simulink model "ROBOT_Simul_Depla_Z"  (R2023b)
settings: Solver=ode15s  StartTime=0.0  StopTime=0.2  RelTol=1e-3  EnableMultiTasking=on
undefined symbols (not defined in the file): BATI1_Défaut_sldprt, BATI2_Défaut_sldprt, BATI3_Défaut_sldprt, deg, kg, m, mm, N, rad, s, STL, X, Y, Z
libraries: sm_lib x139, fl_lib x42, nesl_utility x19, slpidlib x3
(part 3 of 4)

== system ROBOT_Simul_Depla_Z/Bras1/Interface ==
  Angular Velocity Source : fl_lib/Mechanical/Mechanical Sources/Ideal Angular Velocity Source
  Torque Sensor : fl_lib/Mechanical/Mechanical Sensors/Ideal Torque Sensor
  C : PMIOPort  Side=Left
  T : PMIOPort  Port=2  Side=Right
  w : PMIOPort  Port=3  Side=Right
  R : PMIOPort  Port=4  Side=Left
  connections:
  R/RConn1 -- Angular Velocity Source/LConn1
  Torque Sensor/LConn1 -- Angular Velocity Source/RConn2
  Torque Sensor/RConn2 -- T/RConn1
  C/RConn1 -- Torque Sensor/RConn1
  Angular Velocity Source/RConn1 -- w/RConn1

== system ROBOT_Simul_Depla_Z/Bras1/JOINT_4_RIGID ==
  ReferenceFrame : sm_lib/Frames and Transforms/Reference Frame
  Solid : sm_lib/Body Elements/File Solid  ExtGeomFileName=\STL\JOINT_Défaut_sldprt.STL  UnitType=Custom  ExtGeomFileUnits=mm  StepReaderType=HEX  ExportConvexHullGeometry=off  InertiaType=Custom  Mass=0.010425088409650831  MassUnits=kg  CenterOfMass=[-2.8413803884081348e-07 7.2198924235006832 8.2870434049836507e-08]  CenterOfMassUnits=mm  MomentsOfInertia=[0.40441054898779027 0.67355736496231777 0.88349580308055875]  MomentsOfInertiaUnits=kg*mm^2  ProductsOfInertia=[5.448486796310623e-10 1.7393207622030534e-07 1.1975376403711247e-08]  ProductsOfInertiaUnits=kg*mm^2  BasedOnType=Density  Density=1000  DensityUnits=kg/(m^3)  DoExposeReferenceFrame=on  SerializedFrames=<Frames/>  GraphicType=FromGeometry  MarkerShape=Sphere  MarkerSize=10  MarkerSizeUnits=m  GraphicVisPropType=SimpleVisualProperties  GraphicDiffuseColor=[0.792156862745098 0.81960784313725488 0.93333333333333335]  GraphicSpecularColor=[0.5 0.5 0.5 1.0]  GraphicAmbientColor=[0.15 0.15 0.15 1.0]  GraphicEmissiveColor=[0.0 0.0 0.0 1.0]  GraphicShininess=75  GraphicOpacity=1
  Transform : sm_lib/Frames and Transforms/Rigid Transform  TranslationMethod=Cartesian  TranslationStandardOffset=0  TranslationStandardOffsetUnits=mm  TranslationStandardAxis=+Z  TranslationCartesianOffset=[13.999999999999849 4.9999999999999574 4.9999999999999956]  TranslationCartesianOffsetUnits=mm  TranslationROffset=0  TranslationROffsetUnits=m  TranslationZOffset=0  TranslationZOffsetUnits=m  TranslationThetaOffset=0  TranslationThetaOffsetUnits=deg  RotationMethod=ArbitraryAxis  RotationAngleUnits=rad  RotationStandardAxis=+Z  RotationAngle=3.1415926535897931  RotationArbitraryAxis=[-1 4.2709310989463294e-33 -8.8869701386798953e-17]  FollAlignAxisA=+X  BaseAlignAxisA=+Y  FollAlignAxisB=+Y  BaseAlignAxisB=+Z  RotationSequenceAxes=FollowerAxes  RotationSequence=XYX  RotationSequenceAngles=[0 0 0]  RotationSequenceAnglesUnits=deg  RotationMatrix=[1 0 0; 0 1 0; 0 0 1]  Quaternion=[1 0 0 0]
  Transform1 : sm_lib/Frames and Transforms/Rigid Transform  TranslationMethod=Cartesian  TranslationStandardOffset=0  TranslationStandardOffsetUnits=mm  TranslationStandardAxis=+Z  TranslationCartesianOffset=[-14.000000000000142 4.9999999999998455 -4.9999999999999893]  TranslationCartesianOffsetUnits=mm  TranslationROffset=0  TranslationROffsetUnits=m  TranslationZOffset=0  TranslationZOffsetUnits=m  TranslationThetaOffset=0  TranslationThetaOffsetUnits=deg  RotationMethod=ArbitraryAxis  RotationAngleUnits=rad  RotationStandardAxis=+Z  RotationAngle=1.5700924586837749e-16  RotationArbitraryAxis=[-0.99993539825238109 0.011366587959979699 -8.9227205578830452e-19]  FollAlignAxisA=+X  BaseAlignAxisA=+Y  FollAlignAxisB=+Y  BaseAlignAxisB=+Z  RotationSequenceAxes=FollowerAxes  RotationSequence=XYX  RotationSequenceAngles=[0 0 0]  RotationSequenceAnglesUnits=deg  RotationMatrix=[1 0 0; 0 1 0; 0 0 1]  Quaternion=[1 0 0 0]
  Transform2 : sm_lib/Frames and Transforms/Rigid Transform  TranslationMethod=Cartesian  TranslationStandardOffset=0  TranslationStandardOffsetUnits=mm  TranslationStandardAxis=+Z  TranslationCartesianOffset=[-9.9999999999997335 16.250000000000529 -3.0198066269804258e-13]  TranslationCartesianOffsetUnits=mm  TranslationROffset=0  TranslationROffsetUnits=m  TranslationZOffset=0  TranslationZOffsetUnits=m  TranslationThetaOffset=0  TranslationThetaOffsetUnits=deg  RotationMethod=ArbitraryAxis  RotationAngleUnits=rad  RotationStandardAxis=+Z  RotationAngle=2.0943951023931944  RotationArbitraryAxis=[0.57735026918962729 0.57735026918962551 0.57735026918962451]  FollAlignAxisA=+X  BaseAlignAxisA=+Y  FollAlignAxisB=+Y  BaseAlignAxisB=+Z  RotationSequenceAxes=FollowerAxes  RotationSequence=XYX  RotationSequenceAngles=[0 0 0]  RotationSequenceAnglesUnits=deg  RotationMatrix=[1 0 0; 0 1 0; 0 0 1]  Quaternion=[1 0 0 0]
  F2 : PMIOPort  Side=Right
  F1 : PMIOPort  Port=2  Side=Left
  F : PMIOPort  Port=3  Side=Left
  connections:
  Solid/RConn1 -- ReferenceFrame/RConn1 -- Transform/LConn1 -- Transform1/LConn1 -- Transform2/LConn1
  Transform/RConn1 -- F/RConn1
  Transform1/RConn1 -- F1/RConn1
  Transform2/RConn1 -- F2/RConn1

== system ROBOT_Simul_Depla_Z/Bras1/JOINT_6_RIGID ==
  ReferenceFrame : sm_lib/Frames and Transforms/Reference Frame
  Solid : sm_lib/Body Elements/File Solid  ExtGeomFileName=\STL\JOINT_Défaut_sldprt.STL  UnitType=Custom  ExtGeomFileUnits=mm  StepReaderType=HEX  ExportConvexHullGeometry=off  InertiaType=Custom  Mass=0.010425088409650831  MassUnits=kg  CenterOfMass=[-2.8413803884081348e-07 7.2198924235006832 8.2870434049836507e-08]  CenterOfMassUnits=mm  MomentsOfInertia=[0.40441054898779027 0.67355736496231777 0.88349580308055875]  MomentsOfInertiaUnits=kg*mm^2  ProductsOfInertia=[5.448486796310623e-10 1.7393207622030534e-07 1.1975376403711247e-08]  ProductsOfInertiaUnits=kg*mm^2  BasedOnType=Density  Density=1000  DensityUnits=kg/(m^3)  DoExposeReferenceFrame=on  SerializedFrames=<Frames/>  GraphicType=FromGeometry  MarkerShape=Sphere  MarkerSize=10  MarkerSizeUnits=m  GraphicVisPropType=SimpleVisualProperties  GraphicDiffuseColor=[0.792156862745098 0.81960784313725488 0.93333333333333335]  GraphicSpecularColor=[0.5 0.5 0.5 1.0]  GraphicAmbientColor=[0.15 0.15 0.15 1.0]  GraphicEmissiveColor=[0.0 0.0 0.0 1.0]  GraphicShininess=75  GraphicOpacity=1
  Transform : sm_lib/Frames and Transforms/Rigid Transform  TranslationMethod=Cartesian  TranslationStandardOffset=0  TranslationStandardOffsetUnits=mm  TranslationStandardAxis=+Z  TranslationCartesianOffset=[14.000000000000327 5.0000000000000409 -4.9999999999999645]  TranslationCartesianOffsetUnits=mm  TranslationROffset=0  TranslationROffsetUnits=m  TranslationZOffset=0  TranslationZOffsetUnits=m  TranslationThetaOffset=0  TranslationThetaOffsetUnits=deg  RotationMethod=ArbitraryAxis  RotationAngleUnits=rad  RotationStandardAxis=+Z  RotationAngle=2.5476231888929306e-16  RotationArbitraryAxis=[0.25866689172319263 0.96596658282068038 3.1827911693718406e-17]  FollAlignAxisA=+X  BaseAlignAxisA=+Y  FollAlignAxisB=+Y  BaseAlignAxisB=+Z  RotationSequenceAxes=FollowerAxes  RotationSequence=XYX  RotationSequenceAngles=[0 0 0]  RotationSequenceAnglesUnits=deg  RotationMatrix=[1 0 0; 0 1 0; 0 0 1]  Quaternion=[1 0 0 0]
  Transform1 : sm_lib/Frames and Transforms/Rigid Transform  TranslationMethod=Cartesian  TranslationStandardOffset=0  TranslationStandardOffsetUnits=mm  TranslationStandardAxis=+Z  TranslationCartesianOffset=[-13.999999999999677 5.0000000000000444 4.9999999999999964]  TranslationCartesianOffsetUnits=mm  TranslationROffset=0  TranslationROffsetUnits=m  TranslationZOffset=0  TranslationZOffsetUnits=m  TranslationThetaOffset=0  TranslationThetaOffsetUnits=deg  RotationMethod=ArbitraryAxis  RotationAngleUnits=rad  RotationStandardAxis=+Z  RotationAngle=3.1415926535897931  RotationArbitraryAxis=[1 -6.1548272841853811e-33 -8.2569214265266672e-17]  FollAlignAxisA=+X  BaseAlignAxisA=+Y  FollAlignAxisB=+Y  BaseAlignAxisB=+Z  RotationSequenceAxes=FollowerAxes  RotationSequence=XYX  RotationSequenceAngles=[0 0 0]  RotationSequenceAnglesUnits=deg  RotationMatrix=[1 0 0; 0 1 0; 0 0 1]  Quaternion=[1 0 0 0]
  Transform2 : sm_lib/Frames and Transforms/Rigid Transform  TranslationMethod=Cartesian  TranslationStandardOffset=0  TranslationStandardOffsetUnits=mm  TranslationStandardAxis=+Z  TranslationCartesianOffset=[10.000000000006413 16.249999999997939 -2.3288038164537284e-12]  TranslationCartesianOffsetUnits=mm  TranslationROffset=0  TranslationROffsetUnits=m  TranslationZOffset=0  TranslationZOffsetUnits=m  TranslationThetaOffset=0  TranslationThetaOffsetUnits=deg  RotationMethod=ArbitraryAxis  RotationAngleUnits=rad  RotationStandardAxis=+Z  RotationAngle=2.0943951023931966  RotationArbitraryAxis=[-0.5773502691896264 -0.57735026918962618 0.57735026918962484]  FollAlignAxisA=+X  BaseAlignAxisA=+Y  FollAlignAxisB=+Y  BaseAlignAxisB=+Z  RotationSequenceAxes=FollowerAxes  RotationSequence=XYX  RotationSequenceAngles=[0 0 0]  RotationSequenceAnglesUnits=deg  RotationMatrix=[1 0 0; 0 1 0; 0 0 1]  Quaternion=[1 0 0 0]
  F2 : PMIOPort  Side=Left
  F1 : PMIOPort  Port=2  Side=Right
  F : PMIOPort  Port=3  Side=Right
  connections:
  Solid/RConn1 -- ReferenceFrame/RConn1 -- Transform/LConn1 -- Transform1/LConn1 -- Transform2/LConn1
  Transform/RConn1 -- F/RConn1
  Transform1/RConn1 -- F1/RConn1
  Transform2/RConn1 -- F2/RConn1

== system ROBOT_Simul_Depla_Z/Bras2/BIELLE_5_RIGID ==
  ReferenceFrame : sm_lib/Frames and Transforms/Reference Frame
  Solid : sm_lib/Body Elements/File Solid  ExtGeomFileName=\STL\BIELLE_Défaut_sldprt.STL  UnitType=Custom  ExtGeomFileUnits=mm  StepReaderType=HEX  ExportConvexHullGeometry=off  InertiaType=Custom  Mass=0.008350539405564527  MassUnits=kg  CenterOfMass=[0 1.3968069938607398e-07 -5.4963035279888423e-06]  CenterOfMassUnits=mm  MomentsOfInertia=[9.7237898508136684 9.7147278737202658 0.035523108889582884]  MomentsOfInertiaUnits=kg*mm^2  ProductsOfInertia=[0 -4.4011490170351759e-08 -8.1673382975267321e-07]  ProductsOfInertiaUnits=kg*mm^2  BasedOnType=Density  Density=1000  DensityUnits=kg/(m^3)  DoExposeReferenceFrame=on  SerializedFrames=<Frames/>  GraphicType=FromGeometry  MarkerShape=Sphere  MarkerSize=10  MarkerSizeUnits=m  GraphicVisPropType=SimpleVisualProperties  GraphicDiffuseColor=[0.69803921568627447 0.69803921568627447 0.69803921568627447]  GraphicSpecularColor=[0.5 0.5 0.5 1.0]  GraphicAmbientColor=[0.15 0.15 0.15 1.0]  GraphicEmissiveColor=[0.0 0.0 0.0 1.0]  GraphicShininess=75  GraphicOpacity=1
  Transform : sm_lib/Frames and Transforms/Rigid Transform  TranslationMethod=Cartesian  TranslationStandardOffset=0  TranslationStandardOffsetUnits=mm  TranslationStandardAxis=+Z  TranslationCartesianOffset=[0 4.9999999999999973 -51.250000000000007]  TranslationCartesianOffsetUnits=mm  TranslationROffset=0  TranslationROffsetUnits=m  TranslationZOffset=0  TranslationZOffsetUnits=m  TranslationThetaOffset=0  TranslationThetaOffsetUnits=deg  RotationMethod=ArbitraryAxis  RotationAngleUnits=rad  RotationStandardAxis=+Z  RotationAngle=2.0943951023931953  RotationArbitraryAxis=[0.57735026918962584 -0.57735026918962584 0.57735026918962584]  FollAlignAxisA=+X  BaseAlignAxisA=+Y  FollAlignAxisB=+Y  BaseAlignAxisB=+Z  RotationSequenceAxes=FollowerAxes  RotationSequence=XYX  RotationSequenceAngles=[0 0 0]  RotationSequenceAnglesUnits=deg  RotationMatrix=[1 0 0; 0 1 0; 0 0 1]  Quaternion=[1 0 0 0]
  Transform1 : sm_lib/Frames and Transforms/Rigid Transform  TranslationMethod=Cartesian  TranslationStandardOffset=0  TranslationStandardOffsetUnits=mm  TranslationStandardAxis=+Z  TranslationCartesianOffset=[0 5.0000000000000044 51.249999999999993]  TranslationCartesianOffsetUnits=mm  TranslationROffset=0  TranslationROffsetUnits=m  TranslationZOffset=0  TranslationZOffsetUnits=m  TranslationThetaOffset=0  TranslationThetaOffsetUnits=deg  RotationMethod=ArbitraryAxis  RotationAngleUnits=rad  RotationStandardAxis=+Z  RotationAngle=2.0943951023931953  RotationArbitraryAxis=[0.57735026918962584 -0.57735026918962584 0.57735026918962584]  FollAlignAxisA=+X  BaseAlignAxisA=+Y  FollAlignAxisB=+Y  BaseAlignAxisB=+Z  RotationSequenceAxes=FollowerAxes  RotationSequence=XYX  RotationSequenceAngles=[0 0 0]  RotationSequenceAnglesUnits=deg  RotationMatrix=[1 0 0; 0 1 0; 0 0 1]  Quaternion=[1 0 0 0]
  F : PMIOPort  Side=Left
  F1 : PMIOPort  Port=2  Side=Right
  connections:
  Solid/RConn1 -- ReferenceFrame/RConn1 -- Transform/LConn1 -- Transform1/LConn1
  Transform/RConn1 -- F/RConn1
  Transform1/RConn1 -- F1/RConn1

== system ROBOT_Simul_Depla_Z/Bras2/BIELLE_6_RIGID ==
  ReferenceFrame : sm_lib/Frames and Transforms/Reference Frame
  Solid : sm_lib/Body Elements/File Solid  ExtGeomFileName=\STL\BIELLE_Défaut_sldprt.STL  UnitType=Custom  ExtGeomFileUnits=mm  StepReaderType=HEX  ExportConvexHullGeometry=off  InertiaType=Custom  Mass=0.008350539405564527  MassUnits=kg  CenterOfMass=[0 1.3968069938607398e-07 -5.4963035279888423e-06]  CenterOfMassUnits=mm  MomentsOfInertia=[9.7237898508136684 9.7147278737202658 0.035523108889582884]  MomentsOfInertiaUnits=kg*mm^2  ProductsOfInertia=[0 -4.4011490170351759e-08 -8.1673382975267321e-07]  ProductsOfInertiaUnits=kg*mm^2  BasedOnType=Density  Density=1000  DensityUnits=kg/(m^3)  DoExposeReferenceFrame=on  SerializedFrames=<Frames/>  GraphicType=FromGeometry  MarkerShape=Sphere  MarkerSize=10  MarkerSizeUnits=m  GraphicVisPropType=SimpleVisualProperties  GraphicDiffuseColor=[0.69803921568627447 0.69803921568627447 0.69803921568627447]  GraphicSpecularColor=[0.5 0.5 0.5 1.0]  GraphicAmbientColor=[0.15 0.15 0.15 1.0]  GraphicEmissiveColor=[0.0 0.0 0.0 1.0]  GraphicShininess=75  GraphicOpacity=1
  Transform : sm_lib/Frames and Transforms/Rigid Transform  TranslationMethod=Cartesian  TranslationStandardOffset=0  TranslationStandardOffsetUnits=mm  TranslationStandardAxis=+Z  TranslationCartesianOffset=[0 4.9999999999999902 -51.249999999999993]  TranslationCartesianOffsetUnits=mm  TranslationROffset=0  TranslationROffsetUnits=m  TranslationZOffset=0  TranslationZOffsetUnits=m  TranslationThetaOffset=0  TranslationThetaOffsetUnits=deg  RotationMethod=ArbitraryAxis  RotationAngleUnits=rad  RotationStandardAxis=+Z  RotationAngle=2.0943951023931953  RotationArbitraryAxis=[0.57735026918962584 -0.57735026918962584 0.57735026918962584]  FollAlignAxisA=+X  BaseAlignAxisA=+Y  FollAlignAxisB=+Y  BaseAlignAxisB=+Z  RotationSequenceAxes=FollowerAxes  RotationSequence=XYX  RotationSequenceAngles=[0 0 0]  RotationSequenceAnglesUnits=deg  RotationMatrix=[1 0 0; 0 1 0; 0 0 1]  Quaternion=[1 0 0 0]
  Transform1 : sm_lib/Frames and Transforms/Rigid Transform  TranslationMethod=Cartesian  TranslationStandardOffset=0  TranslationStandardOffsetUnits=mm  TranslationStandardAxis=+Z  TranslationCartesianOffset=[0 4.9999999999999902 51.25]  TranslationCartesianOffsetUnits=mm  TranslationROffset=0  TranslationROffsetUnits=m  TranslationZOffset=0  TranslationZOffsetUnits=m  TranslationThetaOffset=0  TranslationThetaOffsetUnits=deg  RotationMethod=ArbitraryAxis  RotationAngleUnits=rad  RotationStandardAxis=+Z  RotationAngle=2.0943951023931953  RotationArbitraryAxis=[0.57735026918962584 -0.57735026918962584 0.57735026918962584]  FollAlignAxisA=+X  BaseAlignAxisA=+Y  FollAlignAxisB=+Y  BaseAlignAxisB=+Z  RotationSequenceAxes=FollowerAxes  RotationSequence=XYX  RotationSequenceAngles=[0 0 0]  RotationSequenceAnglesUnits=deg  RotationMatrix=[1 0 0; 0 1 0; 0 0 1]  Quaternion=[1 0 0 0]
  F : PMIOPort  Side=Left
  F1 : PMIOPort  Port=2  Side=Right
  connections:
  Solid/RConn1 -- ReferenceFrame/RConn1 -- Transform/LConn1 -- Transform1/LConn1
  Transform/RConn1 -- F/RConn1
  Transform1/RConn1 -- F1/RConn1

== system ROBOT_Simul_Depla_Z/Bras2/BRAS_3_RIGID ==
  BRAS_1_RIGID : Subsystem
  BRAS_3_RIGID : Subsystem
  ReferenceFrame : sm_lib/Frames and Transforms/Reference Frame
  Transform : sm_lib/Frames and Transforms/Rigid Transform  TranslationMethod=Cartesian  TranslationStandardOffset=0  TranslationStandardOffsetUnits=mm  TranslationStandardAxis=+Z  TranslationCartesianOffset=[-7.3896444519050419e-13 -16.842456388464797 5.0000000000063061]  TranslationCartesianOffsetUnits=mm  TranslationROffset=0  TranslationROffsetUnits=m  TranslationZOffset=0  TranslationZOffsetUnits=m  TranslationThetaOffset=0  TranslationThetaOffsetUnits=deg  RotationMethod=ArbitraryAxis  RotationAngleUnits=rad  RotationStandardAxis=+Z  RotationAngle=3.1415926535897922  RotationArbitraryAxis=[1 -3.4968219954323673e-31 -7.4654377952851924e-16]  FollAlignAxisA=+X  BaseAlignAxisA=+Y  FollAlignAxisB=+Y  BaseAlignAxisB=+Z  RotationSequenceAxes=FollowerAxes  RotationSequence=XYX  RotationSequenceAngles=[0 0 0]  RotationSequenceAnglesUnits=deg  RotationMatrix=[1 0 0; 0 1 0; 0 0 1]  Quaternion=[1 0 0 0]
  Transform1 : sm_lib/Frames and Transforms/Rigid Transform  TranslationMethod=Cartesian  TranslationStandardOffset=0  TranslationStandardOffsetUnits=mm  TranslationStandardAxis=+Z  TranslationCartesianOffset=[0 43.157543611535338 10.000000000006285]  TranslationCartesianOffsetUnits=mm  TranslationROffset=0  TranslationROffsetUnits=m  TranslationZOffset=0  TranslationZOffsetUnits=m  TranslationThetaOffset=0  TranslationThetaOffsetUnits=deg  RotationMethod=ArbitraryAxis  RotationAngleUnits=rad  RotationStandardAxis=+Z  RotationAngle=3.1415926535897931  RotationArbitraryAxis=[1 0 0]  FollAlignAxisA=+X  BaseAlignAxisA=+Y  FollAlignAxisB=+Y  BaseAlignAxisB=+Z  RotationSequenceAxes=FollowerAxes  RotationSequence=XYX  RotationSequenceAngles=[0 0 0]  RotationSequenceAnglesUnits=deg  RotationMatrix=[1 0 0; 0 1 0; 0 0 1]  Quaternion=[1 0 0 0]
  Transform2 : sm_lib/Frames and Transforms/Rigid Transform  TranslationMethod=Cartesian  TranslationStandardOffset=0  TranslationStandardOffsetUnits=mm  TranslationStandardAxis=+Z  TranslationCartesianOffset=[0 -16.842456388464662 6.2762295360840881e-12]  TranslationCartesianOffsetUnits=mm  TranslationROffset=0  TranslationROffsetUnits=m  TranslationZOffset=0  TranslationZOffsetUnits=m  TranslationThetaOffset=0  TranslationThetaOffsetUnits=deg  RotationMethod=None  RotationAngleUnits=deg  RotationStandardAxis=+Z  RotationAngle=0  RotationArbitraryAxis=[0 0 1]  FollAlignAxisA=+X  BaseAlignAxisA=+Y  FollAlignAxisB=+Y  BaseAlignAxisB=+Z  RotationSequenceAxes=FollowerAxes  RotationSequence=XYX  RotationSequenceAngles=[0 0 0]  RotationSequenceAnglesUnits=deg  RotationMatrix=[1 0 0; 0 1 0; 0 0 1]  Quaternion=[1 0 0 0]
  Transform3 : sm_lib/Frames and Transforms/Rigid Transform  TranslationMethod=Cartesian  TranslationStandardOffset=0  TranslationStandardOffsetUnits=mm  TranslationStandardAxis=+Z  TranslationCartesianOffset=[0 43.157543611535338 6.2692906421801808e-12]  TranslationCartesianOffsetUnits=mm  TranslationROffset=0  TranslationROffsetUnits=m  TranslationZOffset=0  TranslationZOffsetUnits=m  TranslationThetaOffset=0  TranslationThetaOffsetUnits=deg  RotationMethod=ArbitraryAxis  RotationAngleUnits=rad  RotationStandardAxis=+Z  RotationAngle=3.1415926535897931  RotationArbitraryAxis=[0 0 1]  FollAlignAxisA=+X  BaseAlignAxisA=+Y  FollAlignAxisB=+Y  BaseAlignAxisB=+Z  RotationSequenceAxes=FollowerAxes  RotationSequence=XYX  RotationSequenceAngles=[0 0 0]  RotationSequenceAnglesUnits=deg  RotationMatrix=[1 0 0; 0 1 0; 0 0 1]  Quaternion=[1 0 0 0]
  F : PMIOPort  Side=Left
  F1 : PMIOPort  Port=2  Side=Right
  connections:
  Transform/LConn1 -- ReferenceFrame/RConn1 -- Transform1/LConn1 -- Transform2/LConn1 -- Transform3/LConn1
  Transform/RConn1 -- F/RConn1
  Transform1/RConn1 -- F1/RConn1
  BRAS_1_RIGID/LConn1 -- Transform2/RConn1
  BRAS_3_RIGID/LConn1 -- Transform3/RConn1

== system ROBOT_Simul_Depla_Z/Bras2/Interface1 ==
  Angular Velocity Source : fl_lib/Mechanical/Mechanical Sources/Ideal Angular Velocity Source
  Torque Sensor : fl_lib/Mechanical/Mechanical Sensors/Ideal Torque Sensor
  C : PMIOPort  Side=Left
  T : PMIOPort  Port=2  Side=Right
  w : PMIOPort  Port=3  Side=Right
  R : PMIOPort  Port=4  Side=Left
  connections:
  Angular Velocity Source/RConn1 -- w/RConn1
  C/RConn1 -- Torque Sensor/RConn1
  Torque Sensor/RConn2 -- T/RConn1
  Torque Sensor/LConn1 -- Angular Velocity Source/RConn2
  R/RConn1 -- Angular Velocity Source/LConn1

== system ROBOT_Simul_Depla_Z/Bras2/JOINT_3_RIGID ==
  ReferenceFrame : sm_lib/Frames and Transforms/Reference Frame
  Solid : sm_lib/Body Elements/File Solid  ExtGeomFileName=\STL\JOINT_Défaut_sldprt.STL  UnitType=Custom  ExtGeomFileUnits=mm  StepReaderType=HEX  ExportConvexHullGeometry=off  InertiaType=Custom  Mass=0.010425088409650831  MassUnits=kg  CenterOfMass=[-2.8413803884081348e-07 7.2198924235006832 8.2870434049836507e-08]  CenterOfMassUnits=mm  MomentsOfInertia=[0.40441054898779027 0.67355736496231777 0.88349580308055875]  MomentsOfInertiaUnits=kg*mm^2  ProductsOfInertia=[5.448486796310623e-10 1.7393207622030534e-07 1.1975376403711247e-08]  ProductsOfInertiaUnits=kg*mm^2  BasedOnType=Density  Density=1000  DensityUnits=kg/(m^3)  DoExposeReferenceFrame=on  SerializedFrames=<Frames/>  GraphicType=FromGeometry  MarkerShape=Sphere  MarkerSize=10  MarkerSizeUnits=m  GraphicVisPropType=SimpleVisualProperties  GraphicDiffuseColor=[0.792156862745098 0.81960784313725488 0.93333333333333335]  GraphicSpecularColor=[0.5 0.5 0.5 1.0]  GraphicAmbientColor=[0.15 0.15 0.15 1.0]  GraphicEmissiveColor=[0.0 0.0 0.0 1.0]  GraphicShininess=75  GraphicOpacity=1
  Transform : sm_lib/Frames and Transforms/Rigid Transform  TranslationMethod=Cartesian  TranslationStandardOffset=0  TranslationStandardOffsetUnits=mm  TranslationStandardAxis=+Z  TranslationCartesianOffset=[14.000000000000393 5.0000000000002949 4.9999999999999307]  TranslationCartesianOffsetUnits=mm  TranslationROffset=0  TranslationROffsetUnits=m  TranslationZOffset=0  TranslationZOffsetUnits=m  TranslationThetaOffset=0  TranslationThetaOffsetUnits=deg  RotationMethod=ArbitraryAxis  RotationAngleUnits=rad  RotationStandardAxis=+Z  RotationAngle=3.1415926535897927  RotationArbitraryAxis=[1 2.4716035461156956e-31 6.8614764825058098e-16]  FollAlignAxisA=+X  BaseAlignAxisA=+Y  FollAlignAxisB=+Y  BaseAlignAxisB=+Z  RotationSequenceAxes=FollowerAxes  RotationSequence=XYX  RotationSequenceAngles=[0 0 0]  RotationSequenceAnglesUnits=deg  RotationMatrix=[1 0 0; 0 1 0; 0 0 1]  Quaternion=[1 0 0 0]
  Transform1 : sm_lib/Frames and Transforms/Rigid Transform  TranslationMethod=Cartesian  TranslationStandardOffset=0  TranslationStandardOffsetUnits=mm  TranslationStandardAxis=+Z  TranslationCartesianOffset=[-13.999999999999581 5.0000000000001972 4.9999999999999769]  TranslationCartesianOffsetUnits=mm  TranslationROffset=0  TranslationROffsetUnits=m  TranslationZOffset=0  TranslationZOffsetUnits=m  TranslationThetaOffset=0  TranslationThetaOffsetUnits=deg  RotationMethod=ArbitraryAxis  RotationAngleUnits=rad  RotationStandardAxis=+Z  RotationAngle=3.1415926535897931  RotationArbitraryAxis=[1 6.1605098685514057e-33 4.1234572726680469e-16]  FollAlignAxisA=+X  BaseAlignAxisA=+Y  FollAlignAxisB=+Y  BaseAlignAxisB=+Z  RotationSequenceAxes=FollowerAxes  RotationSequence=XYX  RotationSequenceAngles=[0 0 0]  RotationSequenceAnglesUnits=deg  RotationMatrix=[1 0 0; 0 1 0; 0 0 1]  Quaternion=[1 0 0 0]
  Transform2 : sm_lib/Frames and Transforms/Rigid Transform  TranslationMethod=Cartesian  TranslationStandardOffset=0  TranslationStandardOffsetUnits=mm  TranslationStandardAxis=+Z  TranslationCartesianOffset=[-10.000000000000021 16.250000000001698 1.8616219676914625e-12]  TranslationCartesianOffsetUnits=mm  TranslationROffset=0  TranslationROffsetUnits=m  TranslationZOffset=0  TranslationZOffsetUnits=m  TranslationThetaOffset=0  TranslationThetaOffsetUnits=deg  RotationMethod=ArbitraryAxis  RotationAngleUnits=rad  RotationStandardAxis=+Z  RotationAngle=2.0943951023931962  RotationArbitraryAxis=[0.57735026918962506 0.57735026918962606 0.57735026918962606]  FollAlignAxisA=+X  BaseAlignAxisA=+Y  FollAlignAxisB=+Y  BaseAlignAxisB=+Z  RotationSequenceAxes=FollowerAxes  RotationSequence=XYX  RotationSequenceAngles=[0 0 0]  RotationSequenceAnglesUnits=deg  RotationMatrix=[1 0 0; 0 1 0; 0 0 1]  Quaternion=[1 0 0 0]
  F2 : PMIOPort  Side=Left
  F1 : PMIOPort  Port=2  Side=Right
  F : PMIOPort  Port=3  Side=Right
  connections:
  Solid/RConn1 -- ReferenceFrame/RConn1 -- Transform/LConn1 -- Transform1/LConn1 -- Transform2/LConn1
  Transform/RConn1 -- F/RConn1
  Transform1/RConn1 -- F1/RConn1
  Transform2/RConn1 -- F2/RConn1

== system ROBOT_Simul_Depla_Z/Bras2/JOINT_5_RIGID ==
  ReferenceFrame : sm_lib/Frames and Transforms/Reference Frame
  Solid : sm_lib/Body Elements/File Solid  ExtGeomFileName=\STL\JOINT_Défaut_sldprt.STL  UnitType=Custom  ExtGeomFileUnits=mm  StepReaderType=HEX  ExportConvexHullGeometry=off  InertiaType=Custom  Mass=0.010425088409650831  MassUnits=kg  CenterOfMass=[-2.8413803884081348e-07 7.2198924235006832 8.2870434049836507e-08]  CenterOfMassUnits=mm  MomentsOfInertia=[0.40441054898779027 0.67355736496231777 0.88349580308055875]  MomentsOfInertiaUnits=kg*mm^2  ProductsOfInertia=[5.448486796310623e-10 1.7393207622030534e-07 1.1975376403711247e-08]  ProductsOfInertiaUnits=kg*mm^2  BasedOnType=Density  Density=1000  DensityUnits=kg/(m^3)  DoExposeReferenceFrame=on  SerializedFrames=<Frames/>  GraphicType=FromGeometry  MarkerShape=Sphere  MarkerSize=10  MarkerSizeUnits=m  GraphicVisPropType=SimpleVisualProperties  GraphicDiffuseColor=[0.792156862745098 0.81960784313725488 0.93333333333333335]  GraphicSpecularColor=[0.5 0.5 0.5 1.0]  GraphicAmbientColor=[0.15 0.15 0.15 1.0]  GraphicEmissiveColor=[0.0 0.0 0.0 1.0]  GraphicShininess=75  GraphicOpacity=1
  Transform : sm_lib/Frames and Transforms/Rigid Transform  TranslationMethod=Cartesian  TranslationStandardOffset=0  TranslationStandardOffsetUnits=mm  TranslationStandardAxis=+Z  TranslationCartesianOffset=[-13.99999999999973 4.9999999999999307 4.9999999999999662]  TranslationCartesianOffsetUnits=mm  TranslationROffset=0  TranslationROffsetUnits=m  TranslationZOffset=0  TranslationZOffsetUnits=m  TranslationThetaOffset=0  TranslationThetaOffsetUnits=deg  RotationMethod=ArbitraryAxis  RotationAngleUnits=rad  RotationStandardAxis=+Z  RotationAngle=3.1415926535897931  RotationArbitraryAxis=[-1 -6.4240613722994368e-33 4.1034435102868363e-17]  FollAlignAxisA=+X  BaseAlignAxisA=+Y  FollAlignAxisB=+Y  BaseAlignAxisB=+Z  RotationSequenceAxes=FollowerAxes  RotationSequence=XYX  RotationSequenceAngles=[0 0 0]  RotationSequenceAnglesUnits=deg  RotationMatrix=[1 0 0; 0 1 0; 0 0 1]  Quaternion=[1 0 0 0]
  Transform1 : sm_lib/Frames and Transforms/Rigid Transform  TranslationMethod=Cartesian  TranslationStandardOffset=0  TranslationStandardOffsetUnits=mm  TranslationStandardAxis=+Z  TranslationCartesianOffset=[14.000000000000249 4.9999999999997691 4.9999999999999734]  TranslationCartesianOffsetUnits=mm  TranslationROffset=0  TranslationROffsetUnits=m  TranslationZOffset=0  TranslationZOffsetUnits=m  TranslationThetaOffset=0  TranslationThetaOffsetUnits=deg  RotationMethod=ArbitraryAxis  RotationAngleUnits=rad  RotationStandardAxis=+Z  RotationAngle=3.1415926535897927  RotationArbitraryAxis=[1 5.1356244409297584e-32 2.9638105957297091e-16]  FollAlignAxisA=+X  BaseAlignAxisA=+Y  FollAlignAxisB=+Y  BaseAlignAxisB=+Z  RotationSequenceAxes=FollowerAxes  RotationSequence=XYX  RotationSequenceAngles=[0 0 0]  RotationSequenceAnglesUnits=deg  RotationMatrix=[1 0 0; 0 1 0; 0 0 1]  Quaternion=[1 0 0 0]
  Transform2 : sm_lib/Frames and Transforms/Rigid Transform  TranslationMethod=Cartesian  TranslationStandardOffset=0  TranslationStandardOffsetUnits=mm  TranslationStandardAxis=+Z  TranslationCartesianOffset=[10.000000000000179 16.249999999999421 -3.836930773104541e-13]  TranslationCartesianOffsetUnits=mm  TranslationROffset=0  TranslationROffsetUnits=m  TranslationZOffset=0  TranslationZOffsetUnits=m  TranslationThetaOffset=0  TranslationThetaOffsetUnits=deg  RotationMethod=ArbitraryAxis  RotationAngleUnits=rad  RotationStandardAxis=+Z  RotationAngle=2.0943951023931962  RotationArbitraryAxis=[-0.57735026918962651 -0.57735026918962606 0.57735026918962473]  FollAlignAxisA=+X  BaseAlignAxisA=+Y  FollAlignAxisB=+Y  BaseAlignAxisB=+Z  RotationSequenceAxes=FollowerAxes  RotationSequence=XYX  RotationSequenceAngles=[0 0 0]  RotationSequenceAnglesUnits=deg  RotationMatrix=[1 0 0; 0 1 0; 0 0 1]  Quaternion=[1 0 0 0]
  F1 : PMIOPort  Side=Left
  F : PMIOPort  Port=2  Side=Left
  F2 : PMIOPort  Port=3  Side=Right
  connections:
  Solid/RConn1 -- ReferenceFrame/RConn1 -- Transform/LConn1 -- Transform1/LConn1 -- Transform2/LConn1
  Transform/RConn1 -- F/RConn1
  Transform1/RConn1 -- F1/RConn1
  Transform2/RConn1 -- F2/RConn1

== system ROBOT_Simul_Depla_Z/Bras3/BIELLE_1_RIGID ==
  ReferenceFrame : sm_lib/Frames and Transforms/Reference Frame
  Solid : sm_lib/Body Elements/File Solid  ExtGeomFileName=\STL\BIELLE_Défaut_sldprt.STL  UnitType=Custom  ExtGeomFileUnits=mm  StepReaderType=HEX  ExportConvexHullGeometry=off  InertiaType=Custom  Mass=0.008350539405564527  MassUnits=kg  CenterOfMass=[0 1.3968069938607398e-07 -5.4963035279888423e-06]  CenterOfMassUnits=mm  MomentsOfInertia=[9.7237898508136684 9.7147278737202658 0.035523108889582884]  MomentsOfInertiaUnits=kg*mm^2  ProductsOfInertia=[0 -4.4011490170351759e-08 -8.1673382975267321e-07]  ProductsOfInertiaUnits=kg*mm^2  BasedOnType=Density  Density=1000  DensityUnits=kg/(m^3)  DoExposeReferenceFrame=on  SerializedFrames=<Frames/>  GraphicType=FromGeometry  MarkerShape=Sphere  MarkerSize=10  MarkerSizeUnits=m  GraphicVisPropType=SimpleVisualProperties  GraphicDiffuseColor=[0.69803921568627447 0.69803921568627447 0.69803921568627447]  GraphicSpecularColor=[0.5 0.5 0.5 1.0]  GraphicAmbientColor=[0.15 0.15 0.15 1.0]  GraphicEmissiveColor=[0.0 0.0 0.0 1.0]  GraphicShininess=75  GraphicOpacity=1
  Transform : sm_lib/Frames and Transforms/Rigid Transform  TranslationMethod=Cartesian  TranslationStandardOffset=0  TranslationStandardOffsetUnits=mm  TranslationStandardAxis=+Z  TranslationCartesianOffset=[6.4659388954169117e-13 -4.9999999999998401 -51.250000000000263]  TranslationCartesianOffsetUnits=mm  TranslationROffset=0  TranslationROffsetUnits=m  TranslationZOffset=0  TranslationZOffsetUnits=m  TranslationThetaOffset=0  TranslationThetaOffsetUnits=deg  RotationMethod=ArbitraryAxis  RotationAngleUnits=rad  RotationStandardAxis=+Z  RotationAngle=2.0943951023931953  RotationArbitraryAxis=[-0.57735026918962584 -0.57735026918962584 -0.57735026918962584]  FollAlignAxisA=+X  BaseAlignAxisA=+Y  FollAlignAxisB=+Y  BaseAlignAxisB=+Z  RotationSequenceAxes=FollowerAxes  RotationSequence=XYX  RotationSequenceAngles=[0 0 0]  RotationSequenceAnglesUnits=deg  RotationMatrix=[1 0 0; 0 1 0; 0 0 1]  Quaternion=[1 0 0 0]
  Transform1 : sm_lib/Frames and Transforms/Rigid Transform  TranslationMethod=Cartesian  TranslationStandardOffset=0  TranslationStandardOffsetUnits=mm  TranslationStandardAxis=+Z  TranslationCartesianOffset=[0 4.9999999999999973 51.249999999999986]  TranslationCartesianOffsetUnits=mm  TranslationROffset=0  TranslationROffsetUnits=m  TranslationZOffset=0  TranslationZOffsetUnits=m  TranslationThetaOffset=0  TranslationThetaOffsetUnits=deg  RotationMethod=ArbitraryAxis  RotationAngleUnits=rad  RotationStandardAxis=+Z  RotationAngle=2.0943951023931953  RotationArbitraryAxis=[0.57735026918962584 -0.57735026918962584 0.57735026918962584]  FollAlignAxisA=+X  BaseAlignAxisA=+Y  FollAlignAxisB=+Y  BaseAlignAxisB=+Z  RotationSequenceAxes=FollowerAxes  RotationSequence=XYX  RotationSequenceAngles=[0 0 0]  RotationSequenceAnglesUnits=deg  RotationMatrix=[1 0 0; 0 1 0; 0 0 1]  Quaternion=[1 0 0 0]
  F : PMIOPort  Side=Left
  F1 : PMIOPort  Port=2  Side=Right
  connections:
  Solid/RConn1 -- ReferenceFrame/RConn1 -- Transform/LConn1 -- Transform1/LConn1
  Transform/RConn1 -- F/RConn1
  Transform1/RConn1 -- F1/RConn1

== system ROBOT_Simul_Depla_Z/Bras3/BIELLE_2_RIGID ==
  ReferenceFrame : sm_lib/Frames and Transforms/Reference Frame
  Solid : sm_lib/Body Elements/File Solid  ExtGeomFileName=\STL\BIELLE_Défaut_sldprt.STL  UnitType=Custom  ExtGeomFileUnits=mm  StepReaderType=HEX  ExportConvexHullGeometry=off  InertiaType=Custom  Mass=0.008350539405564527  MassUnits=kg  CenterOfMass=[0 1.3968069938607398e-07 -5.4963035279888423e-06]  CenterOfMassUnits=mm  MomentsOfInertia=[9.7237898508136684 9.7147278737202658 0.035523108889582884]  MomentsOfInertiaUnits=kg*mm^2  ProductsOfInertia=[0 -4.4011490170351759e-08 -8.1673382975267321e-07]  ProductsOfInertiaUnits=kg*mm^2  BasedOnType=Density  Density=1000  DensityUnits=kg/(m^3)  DoExposeReferenceFrame=on  SerializedFrames=<Frames/>  GraphicType=FromGeometry  MarkerShape=Sphere  MarkerSize=10  MarkerSizeUnits=m  GraphicVisPropType=SimpleVisualProperties  GraphicDiffuseColor=[0.69803921568627447 0.69803921568627447 0.69803921568627447]  GraphicSpecularColor=[0.5 0.5 0.5 1.0]  GraphicAmbientColor=[0.15 0.15 0.15 1.0]  GraphicEmissiveColor=[0.0 0.0 0.0 1.0]  GraphicShininess=75  GraphicOpacity=1
  Transform : sm_lib/Frames and Transforms/Rigid Transform  TranslationMethod=Cartesian  TranslationStandardOffset=0  TranslationStandardOffsetUnits=mm  TranslationStandardAxis=+Z  TranslationCartesianOffset=[-6.5369931689929217e-13 -5.0000000000000746 51.250000000000604]  TranslationCartesianOffsetUnits=mm  TranslationROffset=0  TranslationROffsetUnits=m  TranslationZOffset=0  TranslationZOffsetUnits=m  TranslationThetaOffset=0  TranslationThetaOffsetUnits=deg  RotationMethod=ArbitraryAxis  RotationAngleUnits=rad  RotationStandardAxis=+Z  RotationAngle=2.0943951023931944  RotationArbitraryAxis=[-0.5773502691896254 -0.57735026918962551 -0.5773502691896264]  FollAlignAxisA=+X  BaseAlignAxisA=+Y  FollAlignAxisB=+Y  BaseAlignAxisB=+Z  RotationSequenceAxes=FollowerAxes  RotationSequence=XYX  RotationSequenceAngles=[0 0 0]  RotationSequenceAnglesUnits=deg  RotationMatrix=[1 0 0; 0 1 0; 0 0 1]  Quaternion=[1 0 0 0]
  Transform1 : sm_lib/Frames and Transforms/Rigid Transform  TranslationMethod=Cartesian  TranslationStandardOffset=0  TranslationStandardOffsetUnits=mm  TranslationStandardAxis=+Z  TranslationCartesianOffset=[0 4.9999999999999902 -51.250000000000007]  TranslationCartesianOffsetUnits=mm  TranslationROffset=0  TranslationROffsetUnits=m  TranslationZOffset=0  TranslationZOffsetUnits=m  TranslationThetaOffset=0  TranslationThetaOffsetUnits=deg  RotationMethod=ArbitraryAxis  RotationAngleUnits=rad  RotationStandardAxis=+Z  RotationAngle=2.0943951023931953  RotationArbitraryAxis=[0.57735026918962584 -0.57735026918962584 0.57735026918962584]  FollAlignAxisA=+X  BaseAlignAxisA=+Y  FollAlignAxisB=+Y  BaseAlignAxisB=+Z  RotationSequenceAxes=FollowerAxes  RotationSequence=XYX  RotationSequenceAngles=[0 0 0]  RotationSequenceAnglesUnits=deg  RotationMatrix=[1 0 0; 0 1 0; 0 0 1]  Quaternion=[1 0 0 0]
  F : PMIOPort  Side=Left
  F1 : PMIOPort  Port=2  Side=Right
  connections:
  Solid/RConn1 -- ReferenceFrame/RConn1 -- Transform/LConn1 -- Transform1/LConn1
  Transform/RConn1 -- F/RConn1
  Transform1/RConn1 -- F1/RConn1

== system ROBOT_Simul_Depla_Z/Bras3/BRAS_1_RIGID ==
  BRAS_1_RIGID : Subsystem
  BRAS_3_RIGID : Subsystem
  ReferenceFrame : sm_lib/Frames and Transforms/Reference Frame
  Transform : sm_lib/Frames and Transforms/Rigid Transform  TranslationMethod=Cartesian  TranslationStandardOffset=0  TranslationStandardOffsetUnits=mm  TranslationStandardAxis=+Z  TranslationCartesianOffset=[0 -16.842456388464662 10.000000000006278]  TranslationCartesianOffsetUnits=mm  TranslationROffset=0  TranslationROffsetUnits=m  TranslationZOffset=0  TranslationZOffsetUnits=m  TranslationThetaOffset=0  TranslationThetaOffsetUnits=deg  RotationMethod=ArbitraryAxis  RotationAngleUnits=rad  RotationStandardAxis=+Z  RotationAngle=3.1415926535897931  RotationArbitraryAxis=[1 0 -1.0717459516511952e-16]  FollAlignAxisA=+X  BaseAlignAxisA=+Y  FollAlignAxisB=+Y  BaseAlignAxisB=+Z  RotationSequenceAxes=FollowerAxes  RotationSequence=XYX  RotationSequenceAngles=[0 0 0]  RotationSequenceAnglesUnits=deg  RotationMatrix=[1 0 0; 0 1 0; 0 0 1]  Quaternion=[1 0 0 0]
  Transform1 : sm_lib/Frames and Transforms/Rigid Transform  TranslationMethod=Cartesian  TranslationStandardOffset=0  TranslationStandardOffsetUnits=mm  TranslationStandardAxis=+Z  TranslationCartesianOffset=[-1.6577693300288846e-15 43.157543611535331 10.000000000006278]  TranslationCartesianOffsetUnits=mm  TranslationROffset=0  TranslationROffsetUnits=m  TranslationZOffset=0  TranslationZOffsetUnits=m  TranslationThetaOffset=0  TranslationThetaOffsetUnits=deg  RotationMethod=ArbitraryAxis  RotationAngleUnits=rad  RotationStandardAxis=+Z  RotationAngle=3.1415926535897931  RotationArbitraryAxis=[1 0 8.2888466501444268e-17]  FollAlignAxisA=+X  BaseAlignAxisA=+Y  FollAlignAxisB=+Y  BaseAlignAxisB=+Z  RotationSequenceAxes=FollowerAxes  RotationSequence=XYX  RotationSequenceAngles=[0 0 0]  RotationSequenceAnglesUnits=deg  RotationMatrix=[1 0 0; 0 1 0; 0 0 1]  Quaternion=[1 0 0 0]
  Transform2 : sm_lib/Frames and Transforms/Rigid Transform  TranslationMethod=Cartesian  TranslationStandardOffset=0  TranslationStandardOffsetUnits=mm  TranslationStandardAxis=+Z  TranslationCartesianOffset=[0 -16.842456388464662 6.2727600891321345e-12]  TranslationCartesianOffsetUnits=mm  TranslationROffset=0  TranslationROffsetUnits=m  TranslationZOffset=0  TranslationZOffsetUnits=m  TranslationThetaOffset=0  TranslationThetaOffsetUnits=deg  RotationMethod=None  RotationAngleUnits=deg  RotationStandardAxis=+Z  RotationAngle=0  RotationArbitraryAxis=[0 0 1]  FollAlignAxisA=+X  BaseAlignAxisA=+Y  FollAlignAxisB=+Y  BaseAlignAxisB=+Z  RotationSequenceAxes=FollowerAxes  RotationSequence=XYX  RotationSequenceAngles=[0 0 0]  RotationSequenceAnglesUnits=deg  RotationMatrix=[1 0 0; 0 1 0; 0 0 1]  Quaternion=[1 0 0 0]
  Transform3 : sm_lib/Frames and Transforms/Rigid Transform  TranslationMethod=Cartesian  TranslationStandardOffset=0  TranslationStandardOffsetUnits=mm  TranslationStandardAxis=+Z  TranslationCartesianOffset=[0 43.157543611535331 6.2831684299879953e-12]  TranslationCartesianOffsetUnits=mm  TranslationROffset=0  TranslationROffsetUnits=m  TranslationZOffset=0  TranslationZOffsetUnits=m  TranslationThetaOffset=0  TranslationThetaOffsetUnits=deg  RotationMethod=ArbitraryAxis  RotationAngleUnits=rad  RotationStandardAxis=+Z  RotationAngle=3.1415926535897931  RotationArbitraryAxis=[-8.2888466501444268e-17 0 1]  FollAlignAxisA=+X  BaseAlignAxisA=+Y  FollAlignAxisB=+Y  BaseAlignAxisB=+Z  RotationSequenceAxes=FollowerAxes  RotationSequence=XYX  RotationSequenceAngles=[0 0 0]  RotationSequenceAnglesUnits=deg  RotationMatrix=[1 0 0; 0 1 0; 0 0 1]  Quaternion=[1 0 0 0]
  F1 : PMIOPort  Side=Right
  F : PMIOPort  Port=2  Side=Left
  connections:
  Transform/LConn1 -- ReferenceFrame/RConn1 -- Transform1/LConn1 -- Transform2/LConn1 -- Transform3/LConn1
  Transform/RConn1 -- F/RConn1
  Transform1/RConn1 -- F1/RConn1
  BRAS_1_RIGID/LConn1 -- Transform2/RConn1
  BRAS_3_RIGID/LConn1 -- Transform3/RConn1

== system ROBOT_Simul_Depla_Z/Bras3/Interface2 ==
  Angular Velocity Source : fl_lib/Mechanical/Mechanical Sources/Ideal Angular Velocity Source
  Torque Sensor : fl_lib/Mechanical/Mechanical Sensors/Ideal Torque Sensor
  C : PMIOPort  Side=Left
  T : PMIOPort  Port=2  Side=Right
  w : PMIOPort  Port=3  Side=Right
  R : PMIOPort  Port=4  Side=Left
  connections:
  R/RConn1 -- Angular Velocity Source/LConn1
  Torque Sensor/LConn1 -- Angular Velocity Source/RConn2
  Torque Sensor/RConn2 -- T/RConn1
  C/RConn1 -- Torque Sensor/RConn1
  Angular Velocity Source/RConn1 -- w/RConn1

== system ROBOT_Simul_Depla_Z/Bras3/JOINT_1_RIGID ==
  ReferenceFrame : sm_lib/Frames and Transforms/Reference Frame
  Solid : sm_lib/Body Elements/File Solid  ExtGeomFileName=\STL\JOINT_Défaut_sldprt.STL  UnitType=Custom  ExtGeomFileUnits=mm  StepReaderType=HEX  ExportConvexHullGeometry=off  InertiaType=Custom  Mass=0.010425088409650831  MassUnits=kg  CenterOfMass=[-2.8413803884081348e-07 7.2198924235006832 8.2870434049836507e-08]  CenterOfMassUnits=mm  MomentsOfInertia=[0.40441054898779027 0.67355736496231777 0.88349580308055875]  MomentsOfInertiaUnits=kg*mm^2  ProductsOfInertia=[5.448486796310623e-10 1.7393207622030534e-07 1.1975376403711247e-08]  ProductsOfInertiaUnits=kg*mm^2  BasedOnType=Density  Density=1000  DensityUnits=kg/(m^3)  DoExposeReferenceFrame=on  SerializedFrames=<Frames/>  GraphicType=FromGeometry  MarkerShape=Sphere  MarkerSize=10  MarkerSizeUnits=m  GraphicVisPropType=SimpleVisualProperties  GraphicDiffuseColor=[0.792156862745098 0.81960784313725488 0.93333333333333335]  GraphicSpecularColor=[0.5 0.5 0.5 1.0]  GraphicAmbientColor=[0.15 0.15 0.15 1.0]  GraphicEmissiveColor=[0.0 0.0 0.0 1.0]  GraphicShininess=75  GraphicOpacity=1
  Transform : sm_lib/Frames and Transforms/Rigid Transform  TranslationMethod=Cartesian  TranslationStandardOffset=0  TranslationStandardOffsetUnits=mm  TranslationStandardAxis=+Z  TranslationCartesianOffset=[-13.999999999999998 5.0000000000000115 5.0000000000000187]  TranslationCartesianOffsetUnits=mm  TranslationROffset=0  TranslationROffsetUnits=m  TranslationZOffset=0  TranslationZOffsetUnits=m  TranslationThetaOffset=0  TranslationThetaOffsetUnits=deg  RotationMethod=ArbitraryAxis  RotationAngleUnits=rad  RotationStandardAxis=+Z  RotationAngle=3.1415926535897931  RotationArbitraryAxis=[1 0 -5.6857825516938873e-17]  FollAlignAxisA=+X  BaseAlignAxisA=+Y  FollAlignAxisB=+Y  BaseAlignAxisB=+Z  RotationSequenceAxes=FollowerAxes  RotationSequence=XYX  RotationSequenceAngles=[0 0 0]  RotationSequenceAnglesUnits=deg  RotationMatrix=[1 0 0; 0 1 0; 0 0 1]  Quaternion=[1 0 0 0]
  Transform1 : sm_lib/Frames and Transforms/Rigid Transform  TranslationMethod=Cartesian  TranslationStandardOffset=0  TranslationStandardOffsetUnits=mm  TranslationStandardAxis=+Z  TranslationCartesianOffset=[14.000000000000009 4.9999999999999973 5.0000000000000044]  TranslationCartesianOffsetUnits=mm  TranslationROffset=0  TranslationROffsetUnits=m  TranslationZOffset=0  TranslationZOffsetUnits=m  TranslationThetaOffset=0  TranslationThetaOffsetUnits=deg  RotationMethod=ArbitraryAxis  RotationAngleUnits=rad  RotationStandardAxis=+Z  RotationAngle=3.1415926535897931  RotationArbitraryAxis=[1 0 -5.6857825516938873e-17]  FollAlignAxisA=+X  BaseAlignAxisA=+Y  FollAlignAxisB=+Y  BaseAlignAxisB=+Z  RotationSequenceAxes=FollowerAxes  RotationSequence=XYX  RotationSequenceAngles=[0 0 0]  RotationSequenceAnglesUnits=deg  RotationMatrix=[1 0 0; 0 1 0; 0 0 1]  Quaternion=[1 0 0 0]
  Transform2 : sm_lib/Frames and Transforms/Rigid Transform  TranslationMethod=Cartesian  TranslationStandardOffset=0  TranslationStandardOffsetUnits=mm  TranslationStandardAxis=+Z  TranslationCartesianOffset=[10.000000000006255 16.249999999999446 5.3290705182007514e-13]  TranslationCartesianOffsetUnits=mm  TranslationROffset=0  TranslationROffsetUnits=m  TranslationZOffset=0  TranslationZOffsetUnits=m  TranslationThetaOffset=0  TranslationThetaOffsetUnits=deg  RotationMethod=ArbitraryAxis  RotationAngleUnits=rad  RotationStandardAxis=+Z  RotationAngle=2.0943951023931953  RotationArbitraryAxis=[-0.57735026918962584 -0.57735026918962562 0.57735026918962595]  FollAlignAxisA=+X  BaseAlignAxisA=+Y  FollAlignAxisB=+Y  BaseAlignAxisB=+Z  RotationSequenceAxes=FollowerAxes  RotationSequence=XYX  RotationSequenceAngles=[0 0 0]  RotationSequenceAnglesUnits=deg  RotationMatrix=[1 0 0; 0 1 0; 0 0 1]  Quaternion=[1 0 0 0]
  F2 : PMIOPort  Side=Left
  F1 : PMIOPort  Port=2  Side=Right
  F : PMIOPort  Port=3  Side=Right
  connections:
  Solid/RConn1 -- ReferenceFrame/RConn1 -- Transform/LConn1 -- Transform1/LConn1 -- Transform2/LConn1
  Transform/RConn1 -- F/RConn1
  Transform1/RConn1 -- F1/RConn1
  Transform2/RConn1 -- F2/RConn1

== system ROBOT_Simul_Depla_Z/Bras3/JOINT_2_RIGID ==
  ReferenceFrame : sm_lib/Frames and Transforms/Reference Frame
  Solid : sm_lib/Body Elements/File Solid  ExtGeomFileName=\STL\JOINT_Défaut_sldprt.STL  UnitType=Custom  ExtGeomFileUnits=mm  StepReaderType=HEX  ExportConvexHullGeometry=off  InertiaType=Custom  Mass=0.010425088409650831  MassUnits=kg  CenterOfMass=[-2.8413803884081348e-07 7.2198924235006832 8.2870434049836507e-08]  CenterOfMassUnits=mm  MomentsOfInertia=[0.40441054898779027 0.67355736496231777 0.88349580308055875]  MomentsOfInertiaUnits=kg*mm^2  ProductsOfInertia=[5.448486796310623e-10 1.7393207622030534e-07 1.1975376403711247e-08]  ProductsOfInertiaUnits=kg*mm^2  BasedOnType=Density  Density=1000  DensityUnits=kg/(m^3)  DoExposeReferenceFrame=on  SerializedFrames=<Frames/>  GraphicType=FromGeometry  MarkerShape=Sphere  MarkerSize=10  MarkerSizeUnits=m  GraphicVisPropType=SimpleVisualProperties  GraphicDiffuseColor=[0.792156862745098 0.81960784313725488 0.93333333333333335]  GraphicSpecularColor=[0.5 0.5 0.5 1.0]  GraphicAmbientColor=[0.15 0.15 0.15 1.0]  GraphicEmissiveColor=[0.0 0.0 0.0 1.0]  GraphicShininess=75  GraphicOpacity=1
  Transform : sm_lib/Frames and Transforms/Rigid Transform  TranslationMethod=Cartesian  TranslationStandardOffset=0  TranslationStandardOffsetUnits=mm  TranslationStandardAxis=+Z  TranslationCartesianOffset=[-13.999999999999371 4.9999999999998597 4.9999999999998881]  TranslationCartesianOffsetUnits=mm  TranslationROffset=0  TranslationROffsetUnits=m  TranslationZOffset=0  TranslationZOffsetUnits=m  TranslationThetaOffset=0  TranslationThetaOffsetUnits=deg  RotationMethod=ArbitraryAxis  RotationAngleUnits=rad  RotationStandardAxis=+Z  RotationAngle=3.1415926535897931  RotationArbitraryAxis=[1 1.6269902822629644e-32 1.2901180678782253e-16]  FollAlignAxisA=+X  BaseAlignAxisA=+Y  FollAlignAxisB=+Y  BaseAlignAxisB=+Z  RotationSequenceAxes=FollowerAxes  RotationSequence=XYX  RotationSequenceAngles=[0 0 0]  RotationSequenceAnglesUnits=deg  RotationMatrix=[1 0 0; 0 1 0; 0 0 1]  Quaternion=[1 0 0 0]
  Transform1 : sm_lib/Frames and Transforms/Rigid Transform  TranslationMethod=Cartesian  TranslationStandardOffset=0  TranslationStandardOffsetUnits=mm  TranslationStandardAxis=+Z  TranslationCartesianOffset=[14.000000000000639 5.0000000000006715 4.9999999999999156]  TranslationCartesianOffsetUnits=mm  TranslationROffset=0  TranslationROffsetUnits=m  TranslationZOffset=0  TranslationZOffsetUnits=m  TranslationThetaOffset=0  TranslationThetaOffsetUnits=deg  RotationMethod=ArbitraryAxis  RotationAngleUnits=rad  RotationStandardAxis=+Z  RotationAngle=3.1415926535897909  RotationArbitraryAxis=[1 -3.616260618277222e-32 -3.0826822740225111e-17]  FollAlignAxisA=+X  BaseAlignAxisA=+Y  FollAlignAxisB=+Y  BaseAlignAxisB=+Z  RotationSequenceAxes=FollowerAxes  RotationSequence=XYX  RotationSequenceAngles=[0 0 0]  RotationSequenceAnglesUnits=deg  RotationMatrix=[1 0 0; 0 1 0; 0 0 1]  Quaternion=[1 0 0 0]
  Transform2 : sm_lib/Frames and Transforms/Rigid Transform  TranslationMethod=Cartesian  TranslationStandardOffset=0  TranslationStandardOffsetUnits=mm  TranslationStandardAxis=+Z  TranslationCartesianOffset=[4.9999999999999973 16.249999999999993 0]  TranslationCartesianOffsetUnits=mm  TranslationROffset=0  TranslationROffsetUnits=m  TranslationZOffset=0  TranslationZOffsetUnits=m  TranslationThetaOffset=0  TranslationThetaOffsetUnits=deg  RotationMethod=ArbitraryAxis  RotationAngleUnits=rad  RotationStandardAxis=+Z  RotationAngle=2.0943951023931953  RotationArbitraryAxis=[-0.57735026918962584 -0.57735026918962584 0.57735026918962584]  FollAlignAxisA=+X  BaseAlignAxisA=+Y  FollAlignAxisB=+Y  BaseAlignAxisB=+Z  RotationSequenceAxes=FollowerAxes  RotationSequence=XYX  RotationSequenceAngles=[0 0 0]  RotationSequenceAnglesUnits=deg  RotationMatrix=[1 0 0; 0 1 0; 0 0 1]  Quaternion=[1 0 0 0]
  F1 : PMIOPort  Side=Left
  F : PMIOPort  Port=2  Side=Left
  F2 : PMIOPort  Port=3  Side=Right
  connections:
  Solid/RConn1 -- ReferenceFrame/RConn1 -- Transform/LConn1 -- Transform1/LConn1 -- Transform2/LConn1
  Transform/RConn1 -- F/RConn1
  Transform1/RConn1 -- F1/RConn1
  Transform2/RConn1 -- F2/RConn1

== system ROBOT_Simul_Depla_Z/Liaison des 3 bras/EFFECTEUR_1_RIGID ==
  ReferenceFrame : sm_lib/Frames and Transforms/Reference Frame
  Solid : sm_lib/Body Elements/File Solid  ExtGeomFileName=\STL\EFFECTEUR_Défaut_sldprt.STL  UnitType=Custom  ExtGeomFileUnits=mm  StepReaderType=HEX  ExportConvexHullGeometry=off  InertiaType=Custom  Mass=0.013453568991832839  MassUnits=kg  CenterOfMass=[-17.212650388480686 -9.9626588451280398 5.5774208666899616]  CenterOfMassUnits=mm  MomentsOfInertia=[1.2849612996466211 1.3154199043910564 2.2338709867359823]  MomentsOfInertiaUnits=kg*mm^2  ProductsOfInertia=[0.035925388048610812 0.056750034506765974 -0.058662844210309435]  ProductsOfInertiaUnits=kg*mm^2  BasedOnType=Density  Density=1000  DensityUnits=kg/(m^3)  DoExposeReferenceFrame=on  SerializedFrames=<Frames/>  GraphicType=FromGeometry  MarkerShape=Sphere  MarkerSize=10  MarkerSizeUnits=m  GraphicVisPropType=SimpleVisualProperties  GraphicDiffuseColor=[0.792156862745098 0.81960784313725488 0.93333333333333335]  GraphicSpecularColor=[0.5 0.5 0.5 1.0]  GraphicAmbientColor=[0.15 0.15 0.15 1.0]  GraphicEmissiveColor=[0.0 0.0 0.0 1.0]  GraphicShininess=75  GraphicOpacity=1
  F : PMIOPort  Side=Left
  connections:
  Solid/RConn1 -- ReferenceFrame/RConn1 -- F/RConn1
